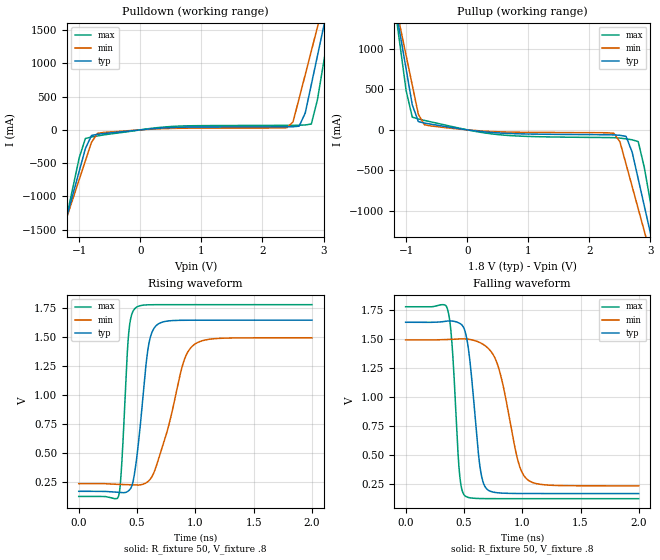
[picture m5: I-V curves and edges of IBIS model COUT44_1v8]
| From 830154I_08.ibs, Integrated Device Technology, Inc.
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[Model] COUT44_1v8
Model_type   Output
Polarity   Non-Inverting
Vmeas = 1.1
Rref = 50
Cref = 0
Vref = .9
|   typ   min   max
C_comp   2pF   1.5pF   2.5pF
|   typ   min   max
[Voltage range]  1.8V   1.710V   1.890V
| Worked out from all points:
|   slope of the pulldown table from 0 to 0.27 V, typ, clamps not added: 12.4 ohm
|   slope of the pullup table from 0 to 0.27 V, typ, clamps not added: 11.3 ohm
|   rising waveform, R_fixture 50, V_fixture .8: 20-80 % time 89.2ps typ, 190ps min, 49.8ps max; typ from 0.167 V to 1.64 V
|   falling waveform, R_fixture 50, V_fixture .8: 20-80 % time 82.4ps typ, 154ps min, 54.6ps max; typ from 1.64 V to 0.167 V
[pulldown]
|Voltage   I (typ)   I (min)   I (max)
-3.3V     -8.339A    -7.182A    -10.24A
-1.3V     -1.626A    -1.582A    -1.703A
-900mV    -280.8mA   -464.6mA   -130.1mA
-700mV    -66.79mA   -52.64mA   -91.41mA
2.4V      45.81mA    32.11mA    67.39mA
2.5V      46.94mA    119.3mA    67.77mA
2.7V      252.9mA    828.7mA    73.03mA
2.8V      682mA      1.186A     87.73mA
2.9V      1.112A     1.544A     453.7mA
3V        1.544A     1.902A     1.005A
3.1V      1.976A     2.261A     1.558A
6.6V      17.45A     15.1A      21.32A
[pullup]
|Voltage   I (typ)   I (min)   I (max)
-3.3V     10.82A     9.291A     13.32A
-1.2V     1.621A     1.64A      1.6A
-1.1V     1.183A     1.277A     1.04A
-900mV    308.9mA    551.5mA    156.6mA
-700mV    83.38mA    62.39mA    116.4mA
2.4V      -62.57mA   -42.43mA   -96.66mA
2.6V      -80.74mA   -420.9mA   -110.7mA
2.8V      -605.9mA   -973.1mA   -144.8mA
2.9V      -939.6mA   -1.25A     -465mA
3V        -1.274A    -1.528A    -892mA
3.1V      -1.609A    -1.806A    -1.319A
6.6V      -13.35A    -11.6A     -16.26A
[Ramp]
|   typ   min   max
dV/dt_r   1.19/.138n   1.01/.281n   1.34/.0774n
dV/dt_f   1.19/.128n   1.01/.249n   1.34/.085n
[Rising Waveform]
R_fixture = 50
V_fixture = .8
V_fixture_max = .945
V_fixture_min = .855
C_fixture = 0.0p
| Time   typ   min   max
0s        167.4mV    233.8mV    123.4mV
342.3ps   158.7mV    227.4mV    129.1mV
367.5ps   156.2mV    226.5mV    383.2mV
428.4ps   172.9mV    223.7mV    1.533V
489.3ps   396.5mV    221.4mV    1.752V
592.2ps   1.386V     250.9mV    1.776V
672ps     1.604V     407.3mV    1.778V
894.6ps   1.643V     1.27V      1.778V
982.8ps   1.644V     1.428V     1.778V
1.999ns   1.644V     1.492V     1.778V
[Falling Waveform]
R_fixture = 50
V_fixture = .8
V_fixture_max = .945
V_fixture_min = .855
C_fixture = 0.0p
| Time   typ   min   max
0s        1.644V     1.492V     1.778V
359.1ps   1.655V     1.495V     1.757V
399ps     1.655V     1.497V     1.441V
462ps     1.636V     1.501V     341.8mV
510.3ps   1.564V     1.5V       147mV
636.3ps   407.5mV    1.469V     124.6mV
697.2ps   205.8mV    1.43V      123.7mV
798ps     173.4mV    1.249V     123.4mV
1.039ns   167.7mV    292.3mV    123.4mV
1.999ns   167.4mV    233.9mV    123.4mV
